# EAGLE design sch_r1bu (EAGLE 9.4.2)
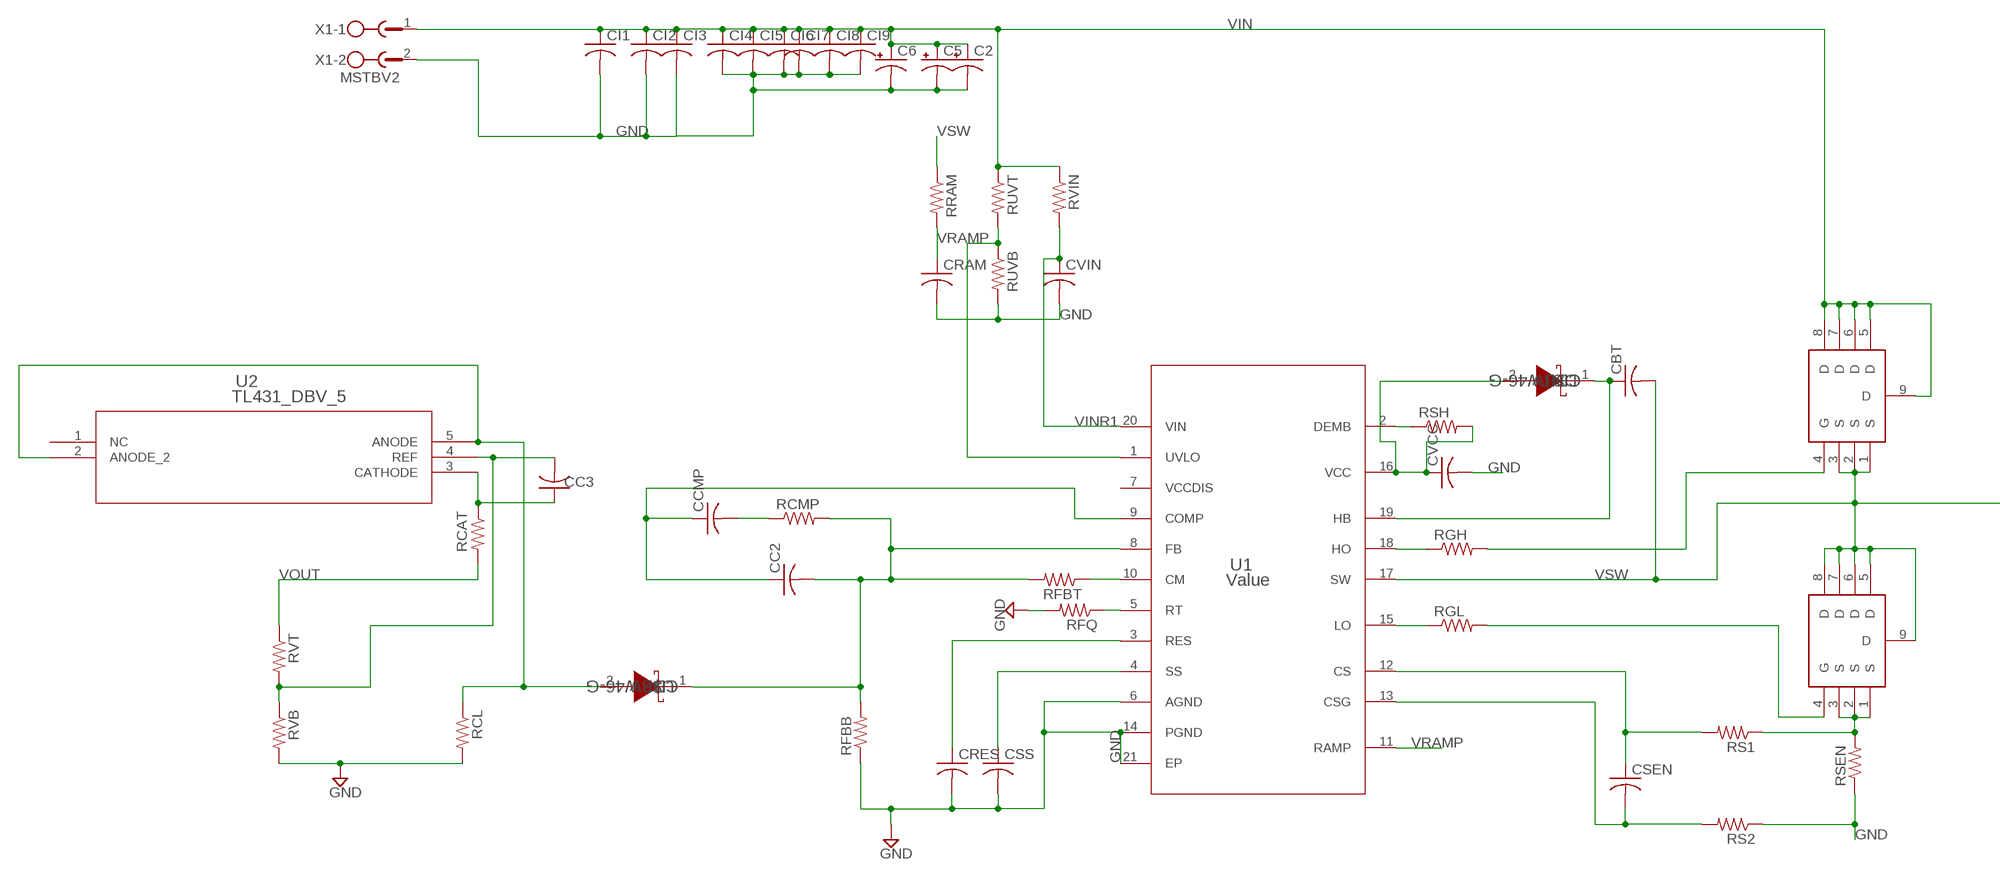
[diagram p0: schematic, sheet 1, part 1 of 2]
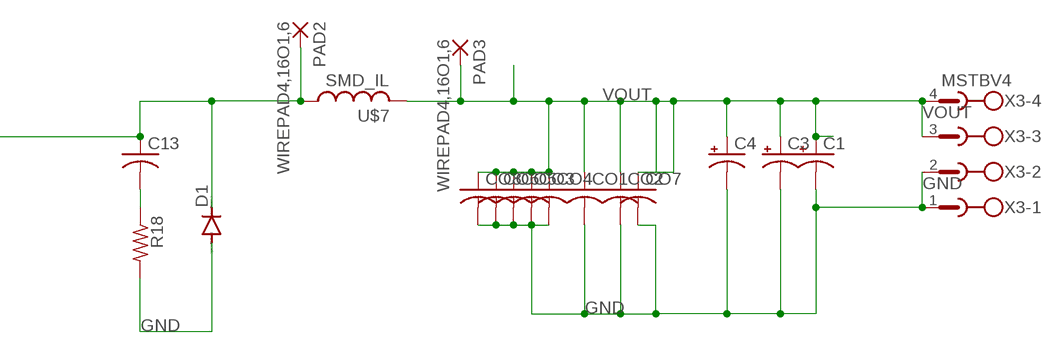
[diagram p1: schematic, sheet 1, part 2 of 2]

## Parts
C1  CPOL-USE5-10.5  [E5-10,5]
C2  CPOL-USE5-10.5  [E5-10,5]
C3  CPOL-USE5-10.5  [E5-10,5]
C4  CPOL-USE5-10.5  [E5-10,5]
C5  CPOL-USE5-10.5  [E5-10,5]
C6  CPOL-USE5-10.5  [E5-10,5]
C13  C-USC1206  [C1206]
CBT  C-USC0603  [C0603]
CC2  C-USC0603  [C0603]
CC3  C-USC0603  [C0603]
CCMP  C-USC0603  [C0603]
CI1  C-USC1206  [C1206]
CI2  C-USC0603  [C0603]
CI3  C-USC1206  [C1206]
CI4  C-USC1206  [C1206]
CI5  C-USC1206  [C1206]
CI6  C-USC1206  [C1206]
CI7  C-USC1206  [C1206]
CI8  C-USC1206  [C1206]
CI9  C-USC1206  [C1206]
CO1  C-USC1206  [C1206]
CO2  C-USC1206  [C1206]
CO3  C-USC1206  [C1206]
CO4  C-USC1206  [C1206]
CO5  C-USC1206  [C1206]
CO6  C-USC1206  [C1206]
CO7  C-USC1206  [C1206]
CO8  C-USC1206  [C1206]
CRAM  C-USC0603  [C0603]
CRES  C-USC0603  [C0603]
CSEN  C-USC0603  [C0603]
CSS  C-USC0603  [C0603]
CVCC  C-USC0603  [C0603]
CVIN  C-USC0603  [C0603]
D1  DIODE-DO214AA  [DO214AA]
DBT  CDBW46-G  [SOD-123]
PAD2  WIREPAD4,16O1,6  [4,16O1,6]
PAD3  WIREPAD4,16O1,6  [4,16O1,6]
R18  R-US_R1206  [R1206]
RCAT  R-US_R0603  [R0603]
RCL  R-US_R0603  [R0603]
RCMP  R-US_R0603  [R0603]
RFBB  R-US_R0603  [R0603]
RFBT  R-US_R0603  [R0603]
RFQ  R-US_R0603  [R0603]
RGH  R-US_R0603  [R0603]
RGL  R-US_R0603  [R0603]
RRAM  R-US_R0603  [R0603]
RS1  R-US_R0603  [R0603]
RS2  R-US_R0603  [R0603]
RSEN  R-US_R3216  [R3216]
RSH  R-US_R0603  [R0603]
RUVB  R-US_R0603  [R0603]
RUVT  R-US_R0603  [R0603]
RVB  R-US_R0603  [R0603]
RVIN  R-US_R0603  [R0603]
RVT  R-US_R0603  [R0603]
U1  Value  LM5117PMHX/NOPB  [PWP0020A]
U2  TL431_DBV_5  [DBV5]
U$2  CDBW46-G  [SOD-123]
U$3  CSD19537Q3  [DQG0008A]
U$4  CSD19537Q3  [DQG0008A]
U$7  SMD_IL  [SMD_ILF]
X1  MSTBV2  [MSTBV2]
X3  MSTBV4  [MSTBV4]

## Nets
GND: C1.- C2.- C3.- C4.- C5.- C6.- CI1.2 CI2.2 CI3.2 CI4.2 CI5.2 CI6.2 CI7.2 CI8.2 CI9.2 CO1.2 CO2.2 CO3.2 CO4.2 CO5.2 CO6.2 CO7.2 CO8.2 CRAM.2 CRES.2 CSS.2 CVCC.2 CVIN.2 D1.A R18.2 RCL.2 RFBB.1 RFQ.2 RS2.1 RSEN.1 RUVB.2 RVB.2 U1.6(AGND) U1.14(PGND) U1.21(EP) X1.2 X3.1 X3.2
N$1: RFQ.1 U1.5(RT)
N$2: RFBT.1 U1.10(CM)
N$3: CRES.1 U1.3(RES)
N$4: CC2.1 CCMP.1 U1.9(COMP)
N$5: CC2.2 RCMP.2 RFBB.2 RFBT.2 U1.8(FB) U$2.1(K)
N$6: CCMP.2 RCMP.1
N$7: RSH.1 U1.2(DEMB)
N$8: CC3.1 RCAT.1 U2.3(CATHODE)
N$9: RUVB.1 RUVT.2 U1.1(UVLO)
N$11: RCL.1 U2.2(ANODE_2) U2.5(ANODE) U$2.2(A)
N$12: CC3.2 RVB.1 RVT.2 U2.4(REF)
N$16: CSS.1 U1.4(SS)
N$19: CSEN.2 RS2.2 U1.13(CSG)
N$20: RGL.2 U$4.4(G)
N$21: RGH.2 U$3.4(G)
N$22: RS1.1 RSEN.2 U$4.1(S) U$4.2(S) U$4.3(S)
N$23: CVCC.1 DBT.2(A) RSH.2 U1.16(VCC)
N$24: CSEN.1 RS1.2 U1.12(CS)
N$25: CBT.1 DBT.1(K) U1.19(HB)
N$27: RGH.1 U1.18(HO)
N$28: C13.2 R18.1
N$30: RGL.1 U1.15(LO)
VIN: C2.+ C5.+ C6.+ CI1.1 CI2.1 CI3.1 CI4.1 CI5.1 CI6.1 CI7.1 CI8.1 CI9.1 RUVT.1 RVIN.1 U$3.5(D) U$3.6(D) U$3.7(D) U$3.8(D) U$3.9(D) X1.1
VINR1: CVIN.1 RVIN.2 U1.20(VIN)
VOUT: C1.+ C3.+ C4.+ CO1.1 CO2.1 CO3.1 CO4.1 CO5.1 CO6.1 CO7.1 CO8.1 PAD3.1(P) RCAT.2 RVT.1 U$7.2 X3.3 X3.4
VRAMP: CRAM.1 RRAM.2 U1.11(RAMP)
VSW: C13.1 CBT.2 D1.C PAD2.1(P) RRAM.1 U1.17(SW) U$3.1(S) U$3.2(S) U$3.3(S) U$4.5(D) U$4.6(D) U$4.7(D) U$4.8(D) U$4.9(D) U$7.1
Unconnected: U1.7(VCCDIS) U2.1(NC)

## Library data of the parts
C1-C6 = rcl:CPOL-US: POLARIZED CAPACITOR, American symbol; SPICEPREFIX: C
C13 CBT CC2 CC3 CCMP CI1-CI9 CO1-CO8 CRAM CRES CSEN CSS CVCC CVIN = rcl:C-US: CAPACITOR, American symbol; SPICEPREFIX: C
D1 = diode:DIODE-: DIODE
DBT U$2 = AcceleratedDesigns_Lib:CDBW46-G; DATASHEETURL: httpwww.comchiptech.comcmsUserFilesCDBW46%2DG%2520RevC.pdf; IO: 0.15; MANUFACTURER_NAME: Comchip Technology; MANUFACTURER_PART_NUMBER: CDBW46G; VENDOR: Comchip Technology; VFATIO: 1.0; VRRM: 100.0
PAD2 PAD3 = wirepad:WIREPAD: Wire PAD connect wire on PCB
R18 RCAT RCL RCMP RFBB RFBT RFQ RGH RGL RRAM RS1 RS2 RSEN RSH RUVB RUVT RVB RVIN RVT = rcl:R-US_: RESISTOR, American symbol; SPICEPREFIX: R
U1 = AcceleratedDesigns_Lib:LM5117PMHX/NOPB; MANUFACTURER: Texas Instruments; MANUFACTURER_NAME: Texas Instruments; MANUFACTURER_PART_NUMBER: LM5117PMHXNOPB; PARTNUMBER: LM5117PMHXNOPB; REFDES: RefDes; TYPE: TYPE
U2 = my_lib:TL431_DBV_5; DATASHEETURL: httpwww.ti.comlitgpnTL431; FAMILY_NAME: SHUNT VOLTAGE REFERENCE; GENERIC_PART_NUMBER: TL431; INDUSTRY_STD_PKG_TYPE: SOT23; MANUFACTURER: Texas Instruments; MANUFACTURER_PART_NUMBER: tl431_dbv_5; PACKAGE_DESIGNATOR: DBV; PIN_COUNT: 5; VENDOR: Texas Instruments
U$3 U$4 = my_lib:CSD19537Q3; DATASHEETURL: httpwww.ti.comlitdssymlinkcsd19537q3.pdf; IDSMAX: 50.0; MANUFACTURER_PART_NUMBER: CSD19537Q3; QGTYP: 16.0; QUANTITY: 1; RDSON45: 0.025; VDSMAX: 100.0; VENDOR: Texas Instruments
U$7 = my_lib:SMD_IL
X1 = con-phoenix-508:MSTBV2: PHOENIX; MPN: MSTBV 2,5/2-GF-5.08; OC_FARNELL: 1792792; OC_NEWARK: 69R9845
X3 = con-phoenix-508:MSTBV4: PHOENIX; MPN: MSTBV 2,5/4-GF-5.08; OC_FARNELL: 1792794; OC_NEWARK: 69R9847

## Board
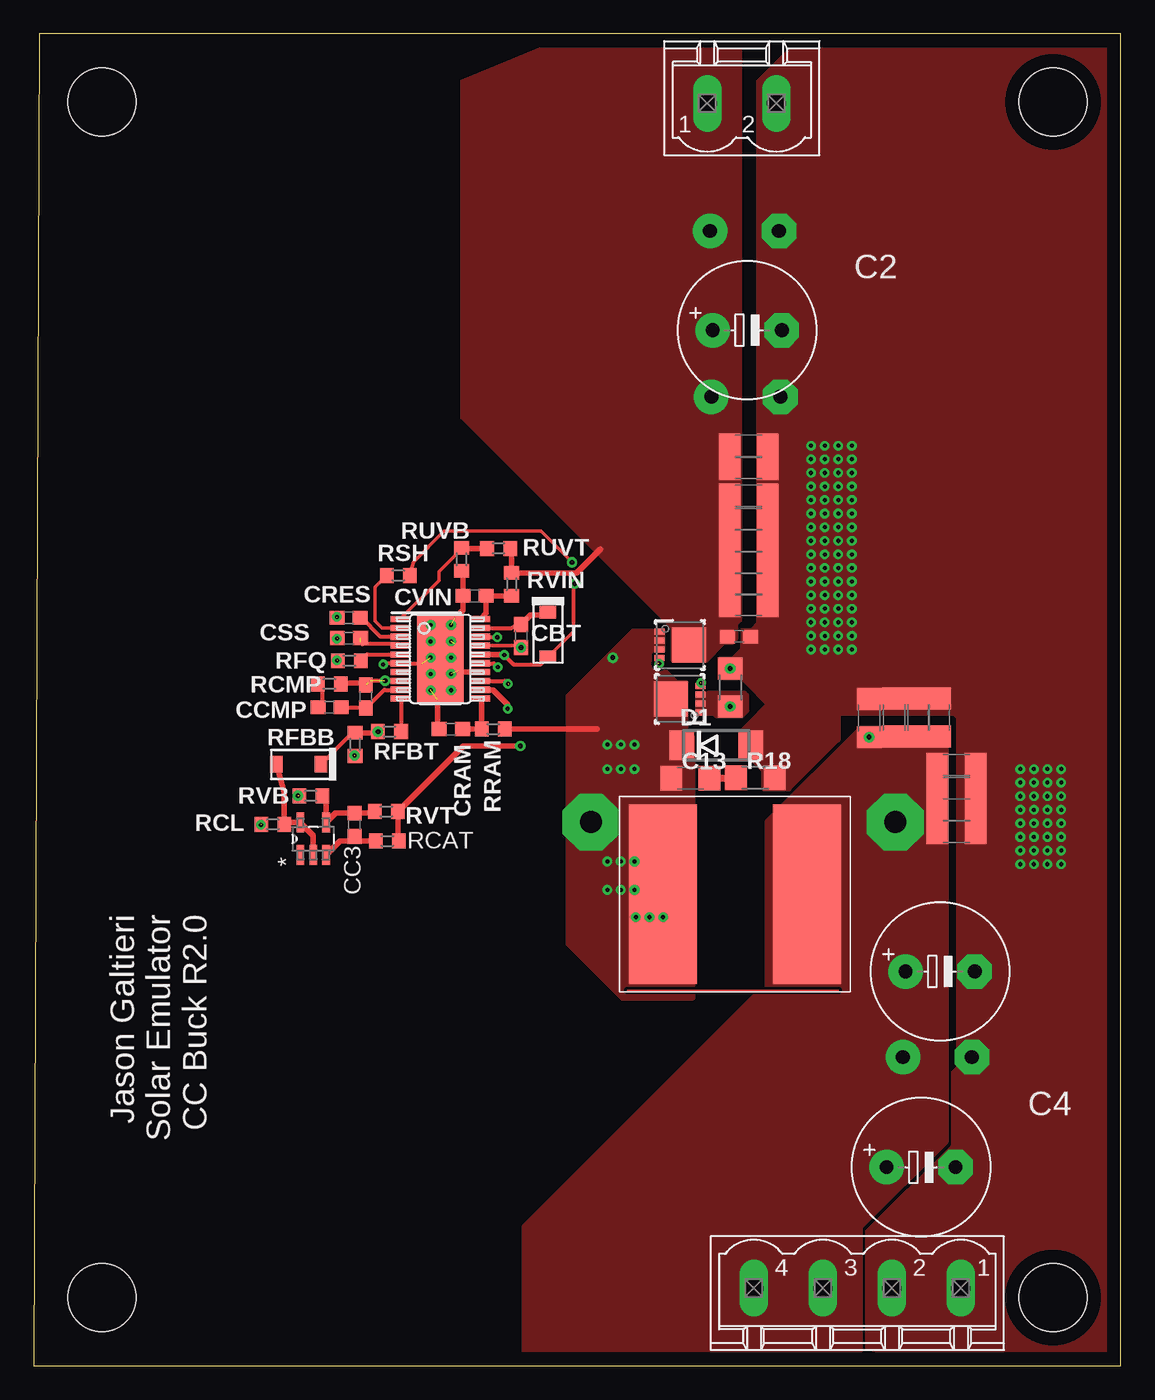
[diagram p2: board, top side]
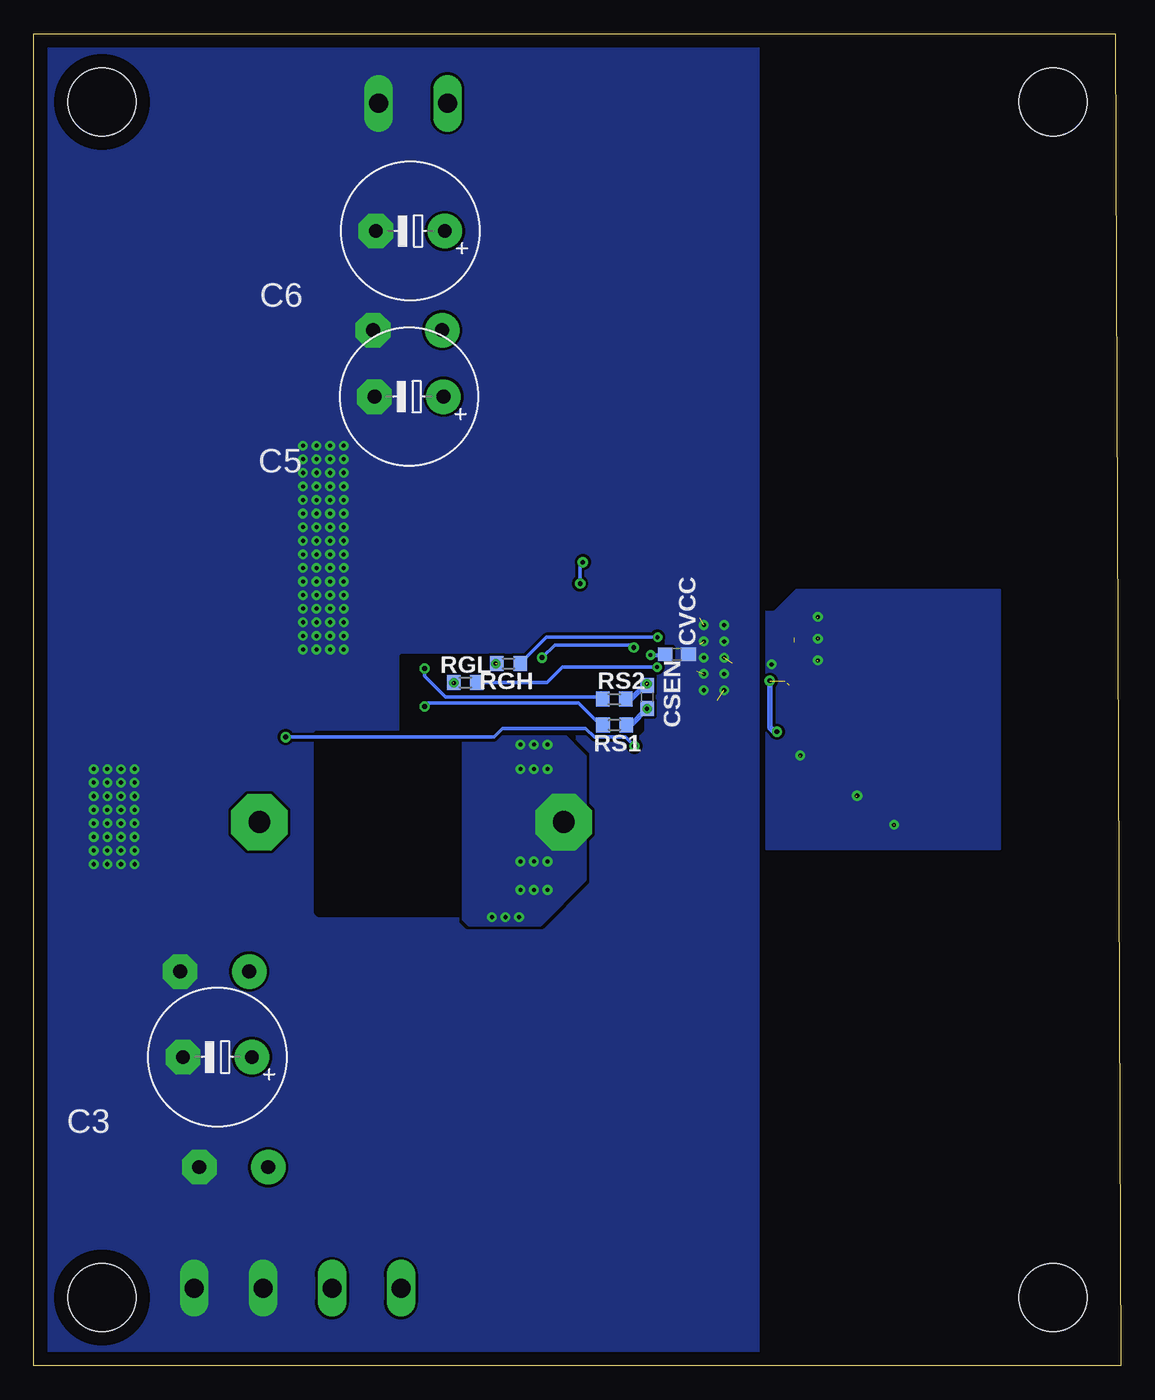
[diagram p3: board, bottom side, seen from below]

Size 80 x 98 mm. Coordinates in mm from the lower left corner, seen from the top.
Outline: 0,0 80,0 80,98 0.4,98 0,0
Copper layers (1*16): Top 0.035mm / dielectric 1.5mm / Bottom 0.035mm
Design rules "default *": minimum track width 6mil, minimum drill 0.35mm, track to track 8mil, track to pad 8mil, pad to pad 8mil, via to via 8mil, smd to smd 6mil, copper to edge 40mil, drill to drill 6mil, minimum pad ring 10mil, minimum via ring 8mil, stop-mask expansion 4mil, vias tented up to drill 0mil, thermal gap 10mil
Holes 5 mm at 5,5 5,93 75,93 75,5

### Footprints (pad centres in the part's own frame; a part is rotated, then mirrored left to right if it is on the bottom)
E5-10,5 = drill 1.016 pad 2.54: + -2.54,0 | drill 1.016 pad 2.54 octagon: - 2.54,0
C1206 = smd 1.6 x 1.8: 1 -1.4,0; 2 1.4,0
C0603 = smd 1.1 x 1: 1 -0.85,0; 2 0.85,0
DO214AA = smd 1.8 x 2.2: A 2.55,0; C -2.55,0
SOD-123 = smd 0.915 x 1.22: 1 -1.637,0; 2 1.637,0
4,16O1,6 = drill 1.6 pad 4.166 octagon: 1 0,0
R1206 = smd 1.6 x 1.803: 1 -1.422,0; 2 1.422,0
R0603 = smd 1 x 1.1: 1 -0.85,0; 2 0.85,0
R3216 = smd 1.6 x 1.8: 1 -1.4,0; 2 1.4,0
PWP0020A = smd 1.4 x 0.45: 1 -2.95,2.925; 2 -2.95,2.275; 3 -2.95,1.625; 4 -2.95,0.975; 5 -2.95,0.325; 6 -2.95,-0.325; 7 -2.95,-0.975; 8 -2.95,-1.625; 9 -2.95,-2.275; 10 -2.95,-2.925; 11 2.95,-2.925; 12 2.95,-2.275; 13 2.95,-1.625; 14 2.95,-0.975; 15 2.95,-0.325; 16 2.95,0.325; 17 2.95,0.975; 18 2.95,1.625; 19 2.95,2.275; 20 2.95,2.925 | smd 3.4 x 6.5: 21 0,0
DBV5 = smd 1.473 x 0.559: 1 -1.194,0.95; 2 -1.194,0; 3 -1.194,-0.95; 4 1.194,-0.95; 5 1.194,0.95
DQG0008A = smd 0.75 x 0.44: 1 -1.525,0.975; 2 -1.525,0.325; 3 -1.525,-0.325; 4 -1.525,-0.975; 5 1.525,-0.975; 6 1.525,-0.325; 7 1.525,0.325; 8 1.525,0.975 | smd 2.5 x 2.55: 9 0.65,0
SMD_ILF = smd 5 x 13.2: 1 0,0; 2 10.6,0
MSTBV2 = drill 1.397 long: 1 -2.54,0; 2 2.54,0
MSTBV4 = drill 1.397 long: 1 -7.62,0; 2 -2.54,0; 3 2.54,0; 4 7.62,0

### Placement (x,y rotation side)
C1  66.7,29 0 top
C2  52.5,76.2 0 top
C3  66.5,22.7 180 bottom
C4  65.3,14.6 0 top
C5  52.4,71.3 180 bottom
C6  52.3,83.5 180 bottom
C13  48.31,43.23 0 top
CBT  35.85,53.69 270 top
CC2  24.44,49.24 90 top
CC3  23.6,39.8 90 top
CCMP  21.75,48.44 180 top
CI1  52.6,66.05 0 top
CI2  51.9,53.65 0 top
CI3  52.6,67.7 0 top
CI4  52.6,64 0 top
CI5  52.6,62.3 0 top
CI6  52.6,60.7 0 top
CI7  52.6,59.1 0 top
CI8  52.6,57.5 0 top
CI9  52.6,56 0 top
CO1  67.9,39.3 0 top
CO2  61.47,47.65 90 top
CO3  65.1,47.7 90 top
CO4  66.6,47.7 90 top
CO5  67.9,44.2 0 top
CO6  67.9,42.5 0 top
CO7  63.3,47.7 90 top
CO8  67.9,40.9 0 top
CRAM  30.68,46.85 180 top
CRES  23.17,55.04 180 top
CSEN  34.87,49.19 90 bottom
CSS  23.18,53.54 180 top
CVCC  32.69,52.35 0 bottom
CVIN  32.44,56.64 180 top
D1  50.21,45.65 0 top
DBT  37.83,53.79 270 top
PAD2  41,40 0 top
PAD3  63.4,40 0 top
R18  53.09,43.25 0 top
RCAT  26,38.6 0 top
RCL  17.58,39.83 180 top
RCMP  21.75,50.17 0 top
RFBB  23.63,45.71 90 top
RFBT  26.17,46.65 180 top
RFQ  23.21,51.87 180 top
RGH  45.07,51.66 180 bottom
RGL  48.25,50.26 180 bottom
RRAM  33.81,46.84 180 top
RS1  37.27,47.14 0 bottom
RS2  37.29,49.04 0 bottom
RSEN  51.25,49.9 270 top
RSH  26.81,58.14 0 top
RUVB  31.47,59.34 270 top
RUVT  34.2,60.14 180 top
RVB  20.37,41.93 180 top
RVIN  35.16,57.49 270 top
RVT  25.94,40.77 180 top
U1  29.91,52.01 0 top
U2  20.55,38.76 90 top
U$2  19.49,44.25 180 top
U$3  47.56,53.03 0 top
U$4  47.52,49.05 180 top
U$7  46.3,34.7 0 top
X1  52.1,92.9 0 top
X3  60.6,5.7 180 top

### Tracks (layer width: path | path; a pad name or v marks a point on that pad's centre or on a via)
GND  (via drill 0.3 pad 0.5, 0.35 pad 0.5)  (11 unrouted)
  Top 0.152: v25.7,51.6 25.67,51.6 25.59,51.69 | 31.27,51.03 31.2,51.1
  Top 0.305: 25.59,51.69 U1.6 28.58,51.69 28.76,51.5 | R18.2 54.06,43.13
  Top 0.406: U1.14 31.27,51.03 | U1.21 31,53.1 | RUVB.2 31.59,58.37 CVIN.2 31.59,55.59 31,55 30.95,55.05 | CRAM.2 29.7,46.98 29.7,49
  Bottom 0.254: RS2.1 38.3,49.2 49.7,49.2 51.25,50.75 RSEN.1
  Bottom 0.406: CVCC.2 31.59,52.1
  other vias: 22.3,51.9 22.3,53.5 22.3,55.1 23.6,44.9 16.7,39.8 72.6,36.9 73.6,36.9 73.6,37.9 72.6,37.9 72.6,38.9 73.6,38.9 73.6,39.9 72.6,39.9 74.6,36.9 75.6,36.9 75.6,37.9 74.6,37.9 74.6,38.9 75.6,38.9 75.6,39.9 74.6,39.9 72.6,40.9 73.6,40.9 73.6,41.9 72.6,41.9 72.6,42.9 73.6,42.9 73.6,43.9 72.6,43.9 74.6,40.9 75.6,40.9 75.6,41.9 74.6,41.9 74.6,42.9 75.6,42.9 75.6,43.9 74.6,43.9 57.2,52.7 58.2,52.7 58.2,53.7 57.2,53.7 57.2,54.7 58.2,54.7 58.2,55.7 57.2,55.7 57.2,56.7 58.2,56.7 58.2,57.7 57.2,57.7 57.2,58.7 58.2,58.7 58.2,59.7 57.2,59.7 59.2,60.7 60.2,60.7 60.2,61.7 59.2,61.7 59.2,62.7 60.2,62.7 60.2,63.7 59.2,63.7 59.2,64.7 60.2,64.7 60.2,65.7 59.2,65.7 59.2,66.7 60.2,66.7 60.2,67.7 59.2,67.7 59.2,52.7 60.2,52.7 60.2,53.7 59.2,53.7 59.2,54.7 60.2,54.7 60.2,55.7 59.2,55.7 59.2,56.7 60.2,56.7 60.2,57.7 59.2,57.7 59.2,58.7 60.2,58.7 60.2,59.7 59.2,59.7 57.2,60.7 58.2,60.7 58.2,61.7 57.2,61.7 57.2,62.7 58.2,62.7 58.2,63.7 57.2,63.7 57.2,64.7 58.2,64.7 58.2,65.7 57.2,65.7 57.2,66.7 58.2,66.7 58.2,67.7 57.2,67.7 29.2,54.5 29.2,53.3 29.2,52.1 29.2,50.9 29.2,49.7 51.25,51.3 30.7,54.5 30.7,53.3 30.7,52.1 30.7,50.9 30.7,49.7 19.42,41.94
  pour Bottom (no thermals): 26.1,38 26.1,55.5 25.5,55.5 23.9,57.1 8.9,57.1 8.9,38
  pour Bottom (rank 2, no thermals): 26.8,0.3 79.8,0.3 79.8,97.7 26.8,97.7
  pour Top (rank 2, no thermals): 52.1,54.1 52.1,52.7 51.4,52 50.5,52 50.5,50.6 52.1,50.6 54.4,48.3 54.4,48 67.7,48 68,47.7 68,21.9 61.2,15.1 61.2,1.29 69.03,-0.26 79.3,0.75 79.3,0.75 79.3,100.3 59.1,100.3 53.3,94.5 53.3,54.6 52.8,54.1
  pour Top (no thermals): 53.8,42.5 53.8,43.8 52.7,44.9 52.1,44.9 52.1,46.6 54.7,49.2 58,49.2 59.1,48.1 59.1,46.1 55.5,42.5
N$1
  Top 0.305: RFQ.1 24.52,52.34 U1.5
N$2
  Top 0.305: U1.10 27.02,49.02 RFBT.1
N$3
  Top 0.305: U1.3 25.52,53.63 24.12,55.04 CRES.1
N$4
  Top 0.305: U1.9 25.79,49.73 CC2.1 24.39,48.44 CCMP.1
N$5  (via drill 0.35 pad 0.5)  (2 unrouted)
  Top 0.305: RFBT.2 25.3,46.67 | RFBB.2 23.51,46.4 | 23.51,46.4 23.63,46.4 | 23.51,46.4 23.28,46.4 U$2.1 | U1.8 24.73,50.38 24.57,50.23
  Top 0.406: 24.57,50.23 23.26,50.23 RCMP.2 | RFBB.2 25.23,46.56 RFBT.2
  Bottom 0.406: RFBT.2 25.52,46.65 25.82,46.95 25.82,50.37 v25.84,50.39
  other vias: 25.32,46.65
N$6
  Top 0.305: CCMP.2 21.22,48.76 21.22,49.85 RCMP.1
N$7
  Top 0.254: RSH.1 25.1,57.28 25.1,56.1 25.1,56 25.1,54.8 25.61,54.28 U1.2
N$8
  Top 0.406: U2.3 22.53,38.6 23.6,38.6 | 23.6,38.6 RCAT.1 | CC3.1 23.6,38.6
N$9
  Top 0.254: U1.1 29.8,57.77 29.8,58.42 31.52,60.14
  Top 0.406: RUVB.1 31.52,60.14 RUVT.2
N$10
  cutout Bottom: 48.7,46.5 48.7,33.2 59,33.2 59.2,33.4 59.2,46.5
N$11
  Top 0.406: U$2.2 18.43,42.17 RCL.1 18.55,39.95 U2.5 20.55,39 U2.2
N$12
  Top 0.406: U2.4 22.22,40.67 23.5,40.67 23.58,40.67 | RVT.2 24.99,40.67 23.58,40.67 | U2.4 21.45,39.95 | U2.4 21.5,41.65 RVB.1 | CC3.2 23.58,40.67
N$16  (1 unrouted)
  Top 0.152: 24.18,53.09 24.03,53.24
  Top 0.305: U1.4 26.86,53.09 24.18,53.09
N$19  (via drill 0.3 pad 0.5)  (1 unrouted)
  Top 0.305: U1.13 34.67,50.38 v34.88,50.18
  Bottom 0.152: 34.94,50.14 34.94,50.11 CSEN.2
  Bottom 0.406: RS2.2 36.04,49.04 34.94,50.14
N$20  (via drill 0.3 pad 0.5)  (1 unrouted)
  Top 0.406: 49.16,50.3 v49.1,50.24 49.05,50.19 U$4.4
N$21  (via drill 0.3 pad 0.5)  (1 unrouted)
  Top 0.406: v46.02,51.66 46.02,52.04 U$3.4
N$22  (via drill 0.35 pad 0.5)
  Bottom 0.254: RS1.1 38.32,47.14 39.92,48.74 51.01,48.74 RSEN.2
  other vias: 51.25,48.5
  pour Top (no thermals): 48.8,49.5 48.8,48 50,48 50.2,47.8 52.1,47.8 52.3,48 52.5,48.2 52.5,49.3 52.3,49.5
N$23  (via drill 0.3 pad 0.5, 0.35 pad 0.5)
  Top 0.254: DBT.2 39.7,54.02 39.7,57.5 39.76,57.55 v39.8,57.55 | v39.6,59.12 37.33,61.4 30.2,61.4 27.94,59.14 RSH.2
  Top 0.305: v34.62,52.29 35.31,51.6 37.28,51.6 DBT.2
  Top 0.406: U1.16 34.57,52.34 v34.62,52.29
  Bottom 0.254: v39.8,57.55 39.8,58.8 39.6,59 v39.6,59.12
  Bottom 0.305: v34.62,52.29 33.6,52.29 CVCC.1
N$24  (via drill 0.3 pad 0.5)
  Top 0.305: 34.87,48.64 CSEN.1
  Top 0.406: U1.12 33.77,49.73 34.87,48.64
  Bottom 0.152: RS1.2 36.07,47.14
  Bottom 0.406: 36.07,47.14 CSEN.1
  other vias: 34.87,48.34
N$25
  Top 0.254: CBT.1 35.44,54.54 35.19,54.28
  Top 0.305: U1.19 35.19,54.28
  Top 0.406: CBT.1 36.54,55.23 37.75,55.23 37.75,55.35 DBT.1
N$27  (via drill 0.3 pad 0.5)
  Top 0.152: 34.1,53.63 v34.1,53.6
  Top 0.305: U1.18 34.1,53.63
  Bottom 0.254: v34.1,53.6 42.28,53.6 RGH.1
N$28
  Top 0.508: C13.2 51.65,43.23 R18.1
N$30  (via drill 0.3 pad 0.5)
  Top 0.305: U1.15 33.86,51.69 v34.14,51.4
  Bottom 0.254: v34.14,51.4 41.1,51.4 42.24,50.26 RGL.1
TT
  cutout Bottom: 35.3,51.4 35.3,46.8 35.5,46.6 52.9,46.6 52.9,52.2 36,52.2 35.3,51.5
VIN
  Top 0.406: 41.7,60.1 39.94,58.34 RVIN.1 35.16,60.03 RUVT.1
  pour Top (no thermals): 47,54.3 47,51.9 49.5,51.9 50.8,53.2 51.4,53.2 51.7,53.5 51.7,54.6 52,54.9 52,97 45.23,98.35 39.44,97.78 31.5,94.49 31.5,69.8
VINR1
  Top 0.152: U1.20
  Top 0.406: U1.20 33.29,55.37 CVIN.1 RVIN.2
VOUT  (via drill 0.35 pad 0.5)
  Top 0.406: RCAT.2 26.79,38.66 RVT.1 31.62,45.6 v35.8,45.6
  Bottom 0.254: CO2.1 46.15,46.25 45.5,46.9 39.4,46.9 38.76,46.26 36.46,46.26 v35.8,45.6
  other vias: 61.47,46.25
  pour Top (no thermals): 67.2,46.9 60.9,46.9 54,40 54,28.1 36.1,10.2 36.1,0.5 60.3,0.5 60.8,1 60.8,10.2 67.1,16.5 67.1,46.8
VRAMP
  Top 0.406: U1.11 32.96,48.98 RRAM.2 CRAM.1
VSW  (via drill 0.3 pad 0.5, 0.35 pad 0.5)
  Top 0.254: U1.17 35.7,52.98 CBT.2
  Top 0.406: RRAM.1 41.44,46.84
  Bottom 0.254: CBT.2 36.05,53.04 41.66,53.04 v42.6,52.1
  other vias: 44.3,33 45.3,33 46.3,33 44.2,35 44.2,37.1 44.2,43.9 43.2,35 42.2,35 42.2,37.1 42.2,43.9 42.2,45.7 43.2,45.7 44.2,45.7 43.2,37.1 43.2,43.9 35.85,52.84
  pour Top (no thermals): 48,50.3 48,46.8 48.5,46.3 48.5,27 43.3,27 39.3,31 39.3,49.3 44.1,54.1 46.3,54.1 46.3,51.3 47.3,50.3
  pour Bottom (no thermals): 48.4,46.3 48.1,46.6 41.3,46.6 39.5,44.8 39.5,35.8 42.8,32.5 47.9,32.5 48.7,33.3

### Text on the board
tNames: Jason Galtieri / Solar Emulator / CC Buck R2.0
